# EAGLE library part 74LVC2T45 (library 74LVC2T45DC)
nexperia, 74LVC2T45, Dual supply translating transceiver, 3-state Source: product page, datasheet
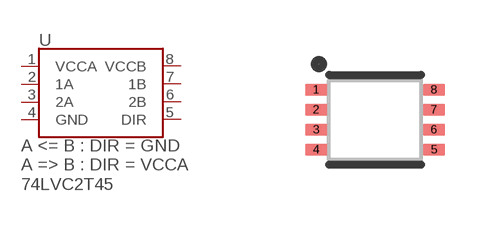
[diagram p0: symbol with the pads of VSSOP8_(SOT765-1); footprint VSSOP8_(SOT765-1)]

Designator prefix U

## 74LVC2T45DC (PROD_ID: IC-19989)  [VSSOP8_(SOT765-1)]
1  VCCA  pwr
2  1A
3  2A
4  GND  pwr
5  DIR  in
6  2B
7  1B
8  VCCB  pwr

## Footprint VSSOP8_(SOT765-1) (pad centres in mm)
VSSOP8 (SOT765-1)
smd 0.55 x 0.3: 1 -1.475,0.75; 2 -1.475,0.25; 3 -1.475,-0.25; 4 -1.475,-0.75; 5 1.475,-0.75; 6 1.475,-0.25; 7 1.475,0.25; 8 1.475,0.75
